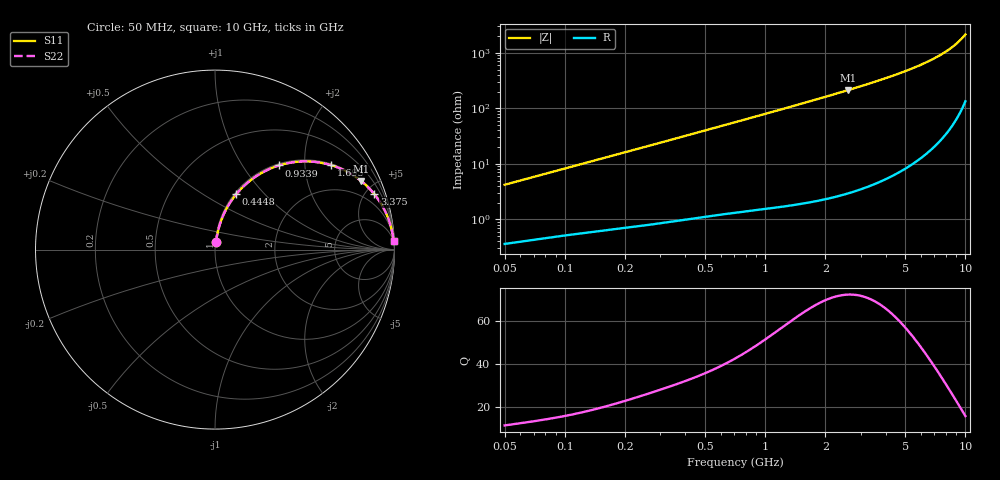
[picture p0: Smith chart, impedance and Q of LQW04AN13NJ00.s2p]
!Murata Part Number: LQW04AN13NJ00
!These Parameters are Measured in Series Mode Connection
!  o--[Z]--o
!Port1  Port2
!  o-------o
!Freq. Start=50[MHz] Stop=10[GHz], 401[Steps]
# Hz S RI R 50
!Freq.(Hz)	S 11(Real)	S 11(Imag)	S 21(Real)	S 21(Imag)	S 12(Real)	S 12(Imag)	S 22(Real)	S 22(Imag)
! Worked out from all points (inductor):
!   401 points, 50 MHz to 10 GHz, reference 50 ohm
!   read as one part in series: L = 13.2 nH near 51.34 MHz
!   highest Q = 72.5 at 2.59 GHz (marker M1), where L = 13 nH
!   S11 on the Smith chart (normalised r, x): 50 MHz: 1.01, +0.08; 444.8 MHz: 1.02, +0.71; 933.9 MHz: 1.03, +1.48; 1.695 GHz: 1.04, +2.71; 3.375 GHz: 1.08, +5.70; 10 GHz: 4, +43
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5e7  0.00532 0.0414  0.9947 -0.0414  0.9947 -0.0414  0.00532 0.0414
1.214486e8  0.0151 0.0969  0.9849 -0.0969  0.9849 -0.0969  0.0151 0.0969
1.930779e8  0.03 0.1499  0.97 -0.1499  0.97 -0.1499  0.03 0.1499
2.949953e8  0.0599 0.2201  0.9401 -0.2201  0.9401 -0.2201  0.0599 0.2201
4.447796e8  0.1185 0.3088  0.8815 -0.3088  0.8815 -0.3088  0.1185 0.3088
5.645355e8  0.1738 0.366  0.8262 -0.366  0.8262 -0.366  0.1738 0.366
7.071068e8  0.2442 0.4181  0.7558 -0.4181  0.7558 -0.4181  0.2442 0.4181
9.338757e8  0.3566 0.469  0.6434 -0.469  0.6434 -0.469  0.3566 0.469
1.26648e9  0.5029 0.4915  0.4971 -0.4915  0.4971 -0.4915  0.5029 0.4915
1.694942e9  0.6454 0.4709  0.3546 -0.4709  0.3546 -0.4709  0.6454 0.4709
1.717543e9  0.6516 0.469  0.3484 -0.469  0.3484 -0.469  0.6516 0.469
2.122994e9  0.7431 0.4299  0.2569 -0.4299  0.2569 -0.4299  0.7431 0.4299
2.589628e9  0.8147 0.3817  0.1853 -0.3817  0.1853 -0.3817  0.8147 0.3817
3.375117e9  0.887 0.3096  0.113 -0.3096  0.113 -0.3096  0.887 0.3096
4.171863e9  0.9277 0.2514  0.0723 -0.2514  0.0723 -0.2514  0.9277 0.2514
5.657692e9  0.9655 0.173  0.0345 -0.173  0.0345 -0.173  0.9655 0.173
7.181012e9  0.9828 0.1172  0.0172 -0.1172  0.0172 -0.1172  0.9828 0.1172
7.878683e9  0.9874 0.0967  0.0126 -0.0967  0.0126 -0.0967  0.9874 0.0967
8.530394e9  0.9906 0.0796  0.00942 -0.0796  0.00942 -0.0796  0.9906 0.0796
9.114482e9  0.9927 0.0656  0.00731 -0.0656  0.00731 -0.0656  0.9927 0.0656
9.738562e9  0.9944 0.0518  0.00563 -0.0518  0.00563 -0.0518  0.9944 0.0518
1e10  0.9949 0.0463  0.00507 -0.0463  0.00507 -0.0463  0.9949 0.0463
